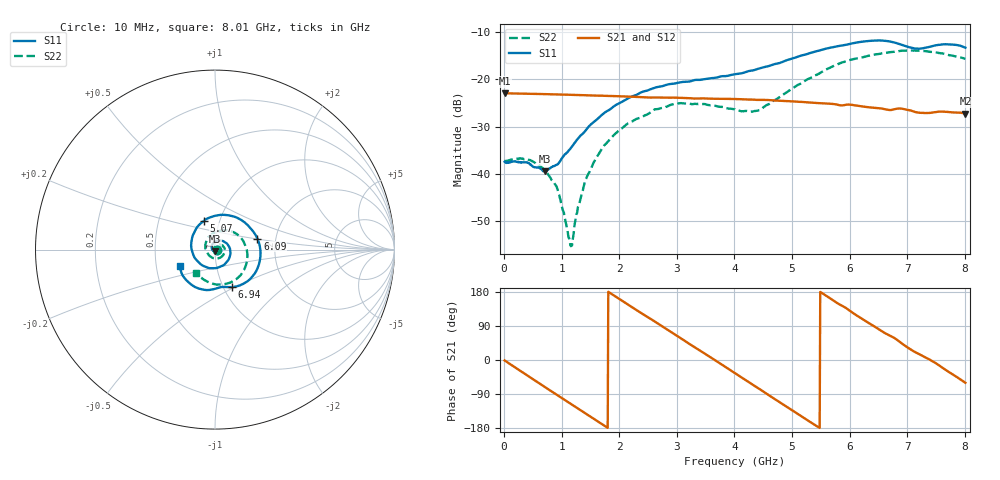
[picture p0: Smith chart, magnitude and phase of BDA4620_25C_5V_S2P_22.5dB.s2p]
!Agilent Technologies,E5071B,MY42404982,A.09.10
!Date: Wed May 06 09:03:13 2026
!Data & Calibration Information:
!Freq	S11:SOLT2(ON)	S21:SOLT2(ON)	S12:SOLT2(ON)	S22:SOLT2(ON)
# Hz S RI R 50
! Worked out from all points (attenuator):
!   801 points, 10 MHz to 8.01 GHz, reference 50 ohm
!   highest |S21| = -22.90 dB at 10 MHz (marker M1); lowest = -27.2 dB at 8.01 GHz (marker M2)
!   lowest |S11| = -39.5 dB at 710 MHz (marker M3), VSWR 1.02, Z = 49.8 - j1.03 ohm
!   |S11| at or under -10 dB: start of sweep to end of sweep
!   |S22| runs from -55.3 to -13.9 dB; largest |S21 - S12| = 0.00031
!   S11 on the Smith chart (normalised r, x): 10 MHz: 1.03, -0.00; 5.07 GHz: 0.84, +0.28; 6.09 GHz: 1.60, +0.21; 6.94 GHz: 1.10, -0.48; 8.01 GHz: 0.66, -0.13
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1e7  0.0134 -0.000887  0.0716 -0.0015  0.0717 -0.00156  0.0137 -0.000476
4.4e8  0.00809 -0.01  0.0504 -0.0494  0.0504 -0.0494  0.0132 -0.00489
7.1e8  -0.00227 -0.0104  0.0223 -0.0663  0.0224 -0.0664  0.00849 -0.00687
9.3e8  -0.0115 -0.00525  -0.00386 -0.0692  -0.00398 -0.0694  0.0034 -0.00592
1.15e9  -0.0175 0.00571  -0.0292 -0.0623  -0.0293 -0.0624  -0.00135 -0.00116
1.19e9  -0.0181 0.00838  -0.0333 -0.06  -0.0335 -0.0601  -0.00199 0.0001
1.26e9  -0.0186 0.013  -0.0402 -0.0554  -0.0403 -0.0555  -0.00306 0.00223
1.35e9  -0.0181 0.0189  -0.0482 -0.0483  -0.0482 -0.0485  -0.0036 0.00501
1.53e9  -0.013 0.0318  -0.0601 -0.0312  -0.0602 -0.0312  -0.00333 0.0116
1.77e9  0.00212 0.0454  -0.0669 -0.00452  -0.067 -0.00452  0.000949 0.0208
2.15e9  0.0396 0.049  -0.055 0.0364  -0.055 0.0365  0.0175 0.0295
2.68e9  0.0835 0.00434  -0.00591 0.0641  -0.00581 0.0641  0.0447 0.0192
3.08e9  0.0762 -0.0544  0.0355 0.0531  0.0356 0.0531  0.0555 -0.00797
4.01e9  -0.0775 -0.0829  0.0509 -0.0354  0.051 -0.0355  -0.0113 -0.047
4.43e9  -0.1307 0.0013  0.0146 -0.059  0.0147 -0.0591  -0.0458 -0.0115
5.07e9  -0.0632 0.1593  -0.0442 -0.038  -0.0445 -0.038  -0.023 0.082
5.35e9  0.0207 0.1923  -0.0552 -0.0129  -0.0553 -0.013  0.0231 0.1032
6.09e9  0.2361 0.0613  -0.0271 0.0457  -0.0273 0.0459  0.1596 0.0438
6.68e9  0.1853 -0.1732  0.0197 0.0432  0.0197 0.0434  0.1706 -0.0911
6.94e9  0.0941 -0.2089  0.0372 0.0312  0.0374 0.0313  0.1372 -0.1481
7.58e9  -0.0797 -0.2197  0.0438 -0.0135  0.0439 -0.0134  -0.0188 -0.1885
8.01e9  -0.1958 -0.0938  0.0217 -0.0377  0.0218 -0.0378  -0.1043 -0.1282
